FUNCTION_BLOCK PusherModule
VAR
	applicationState : I_ApplicationState;
END_VAR

METHOD PUBLIC Execute
VAR_INPUT
END_VAR
VAR
	initSubstate : InitSubstate;
	solenoindExtendSubstate : SolenoindExtendSubstate;
END_VAR
IF applicationState.CurrentState.IsEqual(initSubstate) THEN
	// do what I do to init,
//	applicationSubstate.MoveNext();
	
ELSIF applicationState.CurrentState.IsEqual(solenoindExtendSubstate) THEN
	// do what I do to power on,
	applicationState.MoveNext();
END_IF
END_METHOD

METHOD FB_init : BOOL
VAR_INPUT
	bInitRetains : BOOL; // if TRUE, the retain variables are initialized (warm start / cold start)
	bInCopyCode : BOOL;  // if TRUE, the instance afterwards gets moved into the copy code (online change)
	ApplicationState : I_ApplicationState;
END_VAR
this^.applicationState := ApplicationState;
END_METHOD

END_FUNCTION_BLOCK
